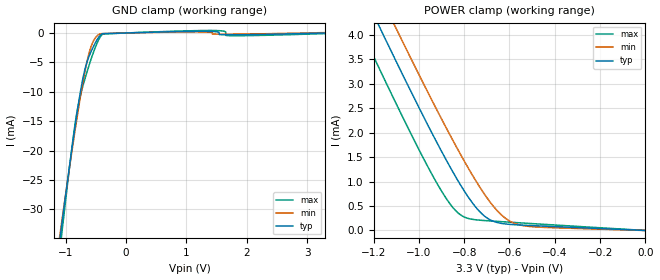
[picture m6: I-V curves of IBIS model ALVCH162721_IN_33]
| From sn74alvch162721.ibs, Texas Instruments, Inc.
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[Model]   ALVCH162721_IN_33
Model_type  Input
Vinl = 0.8
Vinh = 2.0
| variable   typ   min   max
C_comp   1.86pF   1.55pF   2.37pF
[Temperature Range]   40   100   -40
| Ambient temperature   25   85   -40
[Voltage range]   3.3   3   3.6
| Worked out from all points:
|   GND clamp passes 1 mA (typ) near -0.47 V on its own axis
|   POWER clamp passes 1 mA (typ) near -0.83 V on its own axis
[GND Clamp]
| ALVCH162721_IN_33
|   Voltage   I(typ)   I(min)   I(max)
-3.3V     -222.6mA   -207.9mA   -245.6mA
-1.125V   -37.48mA   -36.6mA    -39.69mA
-1.065V   -32.7mA    -32.19mA   -34.28mA
-880mV    -18.51mA   -19.03mA   -18.25mA
-795mV    -12.54mA   -13.36mA   -12.47mA
-700mV    -7.074mA   -7.617mA   -8.518mA
-605mV    -3.802mA   -3.189mA   -5.285mA
-440mV    -556.5uA   -200.5uA   -900.1uA
-375mV    -121.9uA   -99.83uA   -161.9uA
1.165V    276.8uA    180.6uA    398.2uA
1.715V    -314.2uA   -207.1uA   -457.4uA
3.3V      46.64pA    64.32uA    -103.1uA
[POWER Clamp]
| ALVCH162721_IN_33
|   Voltage   I(typ)   I(min)   I(max)
-3.3V     25.56mA    26.05mA    24.96mA
-1.285V   5.237mA    5.897mA    4.391mA
-1.235V   4.75mA     5.413mA    3.898mA
-1.19V    4.314mA    4.981mA    3.457mA
-1.15V    3.929mA    4.598mA    3.068mA
-1.11V    3.547mA    4.218mA    2.683mA
-940mV    1.97mA     2.638mA    1.128mA
-845mV    1.156mA    1.798mA    442.7uA
-725mV    354.6uA    842.3uA    208uA
-625mV    137.3uA    275.3uA    176.9uA
-510mV    102uA      80.87uA    143.3uA
-48.03fV  8.674pA    10.66pA    9.125pA
